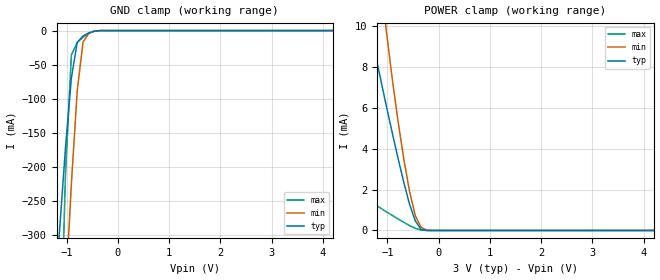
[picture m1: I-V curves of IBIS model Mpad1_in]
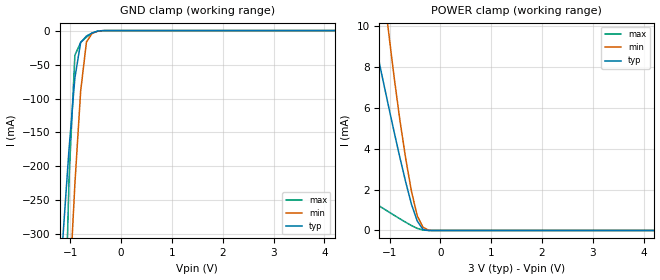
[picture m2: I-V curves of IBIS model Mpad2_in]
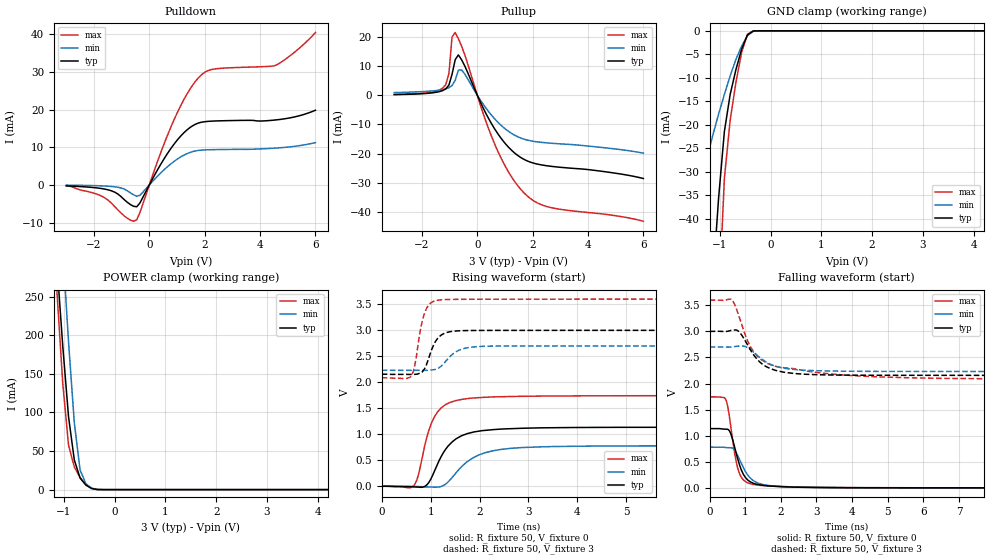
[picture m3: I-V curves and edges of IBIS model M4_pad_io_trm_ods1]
| Created by SiliconSmart  O-2018.09-SP2-3
[IBIS Ver]   4.0
[File Name]   as3316bc_rev1p3.ibs
[File Rev]   1.3
[Date]   Thursday Mar 21 2024
|[Source]   Avalanche Team
|[Notes]   Generated IBIS models from Silicon Smart
|[Rev 1.0]  Initial Release based on extracted netlist
|   Characterization
|[Rev 1.1]  Recharacterization with Hspice, run in high accuracy mode
|[Rev 1.2]  Recharacterization with Hspice, align with datasheet parameter
|[Rev 1.3]  Update the pin to the package pinout assignment
|[Disclaimer]   THE MODEL LIBRARIES ARE PROVIDED AS IS.
|[Copyright]   Copyright 2019, Avalanche Technology., All Rights Reserved
[Component]   as30xx316_BGA
[Manufacturer] Avalanche Technology
| CONTENT :
| This file contains IBIS MODEL for PSRAM device
| AS3001316, AS3004316, AS3008316, AS3016316
| USAGE :
| The models are derived for the 2.7V to 3.6V I/O Operation.
| Temperatures for model generation: typ: 25, max: -40, min: 105
| Voltages : typ: 3.0V, min: 2.7V, max: 3.6V
| PACKAGES SUPPORTED :
| 48-ball FBGA (10mm x 10mm)
| VERIFICATION
| Errors  : 0
| Warnings: 10
| All warnings due to non-monotonic data:
[Package]
R_pkg   0   0 0
L_pkg   0   0 0
C_pkg   0   0 0
[Pin]   signal_name   model_name R_pin   L_pin   C_pin
H6   ADDR_19   Mpad1_in   0.0752   1.401E-09   0.684E-12
H1   ADDR_18   Mpad1_in   0.1092   1.943E-09   0.751E-12
D3   ADDR_17   Mpad1_in   0.1463   2.505E-09   1.065E-12
E4   ADDR_16   Mpad1_in   0.1612   2.777E-09   1.167E-12
F4   ADDR_15   Mpad1_in   0.1337   2.362E-09   1.112E-12
F3   ADDR_14   Mpad1_in   0.1937   3.618E-09   1.182E-12
G4   ADDR_13   Mpad1_in   0.6132   9.666E-09   2.965E-12
G3   ADDR_12   Mpad1_in   0.5553   11.39E-09   2.992E-12
H5   ADDR_11   Mpad1_in   0.5095   10.54E-09   2.784E-12
H4   ADDR_10   Mpad1_in   0.5085   8.139E-09   2.608E-12
H3   ADDR_9   Mpad1_in   0.6314   8.467E-09   2.753E-12
H2   ADDR_8   Mpad1_in   0.6215   8.571E-09   2.739E-12
D4   ADDR_7   Mpad1_in   0.1869   2.994E-09   1.300E-12
C4   ADDR_6   Mpad1_in   0.1507   2.486E-09   1.156E-12
C3   ADDR_5   Mpad1_in   0.1641   2.806E-09   1.081E-12
B4   ADDR_4   Mpad1_in   0.2121   3.648E-09   1.267E-12
B3   ADDR_3   Mpad1_in   0.2174   3.718E-09   1.391E-12
A5   ADDR_2   Mpad1_in   0.2699   5.112E-09   1.665E-12
A4   ADDR_1   Mpad1_in   0.2419   4.762E-09   1.566E-12
A3   ADDR_0   Mpad1_in   0.2438   4.120E-09   1.508E-12
A2   G#   Mpad2_in   0.2799   4.414E-09   1.651E-12
B5   E#   Mpad2_in   0.1988   3.329E-09   1.209E-12
G5   W#   Mpad2_in   0.3304   4.956E-09   1.725E-12
B2   UB#   Mpad2_in   0.3210   5.026E-09   2.051E-12
A1   LB#   Mpad2_in   0.2761   4.637E-09   1.872E-12
G1   DQ_15   Mpad_io   0.0818   1.440E-09   0.758E-12
F1   DQ_14   Mpad_io   0.0722   1.269E-09   0.671E-12
F2   DQ_13   Mpad_io   0.1073   1.763E-09   0.829E-12
E2   DQ_12   Mpad_io   0.1038   1.649E-09   0.806E-12
D2   DQ_11   Mpad_io   0.1029   1.657E-09   0.819E-12
C2   DQ_10   Mpad_io   0.1069   1.768E-09   0.820E-12
C1   DQ_9   Mpad_io   0.0842   1.423E-09   0.731E-12
B1   DQ_8   Mpad_io   0.0865   1.515E-09   0.776E-12
G6   DQ_7   Mpad_io   0.2711   4.295E-09   1.572E-12
F6   DQ_6   Mpad_io   0.1981   3.065E-09   1.253E-12
F5   DQ_5   Mpad_io   0.2781   4.148E-09   1.750E-12
E5   DQ_4   Mpad_io   0.1116   1.847E-09   0.835E-12
D5   DQ_3   Mpad_io   0.1145   1.910E-09   0.901E-12
C6   DQ_2   Mpad_io   0.1632   2.557E-09   1.079E-12
C5   DQ_1   Mpad_io   0.1544   2.582E-09   1.063E-12
B6   DQ_0   Mpad_io   0.2212   3.537E-09   1.114E-12
D1   VSS   GND   NA   NA   NA
E6   VSS   GND   NA   NA   NA
D6   VCC   POWER   NA   NA   NA
E1   VCC   POWER   NA   NA   NA
| pad_io
[Model Selector] Mpad_io
| Model Description
M4_pad_io_trm_ods1   60 Ohms drv strength
| Models and submodels in the file (3): Mpad1_in (Input), Mpad2_in (Input), M4_pad_io_trm_ods1 (I/O)
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| pad1_in
[Model] Mpad1_in
Model_type Input
Enable   Active-High
Vinl  =  0.6
Vinh  =  2.4
| Capacitance  typ   min   max
C_comp   2.857182e-12   2.353202e-12   3.152994e-12
| Variables   typ   min   max
[GND Clamp Reference]   0   0   0
[POWER Clamp Reference]   3   2.7   3.6
[Pulldown Reference]   0   0   0
[Pullup Reference]   3   2.7   3.6
[Temperature Range]   25   105   -40
[Voltage Range]   3   2.7   3.6
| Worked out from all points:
|   GND clamp passes 1 mA (typ) near -0.47 V on its own axis
|   POWER clamp passes 1 mA (typ) near -0.53 V on its own axis
[GND Clamp]
| Voltage   I(typ)   I(min)   I(max)
-3V       -2.489A    -3.622A    -6.286A
-1.252V   -415.1mA   -737.7mA   -841.9mA
-1.138V   -289.6mA   -559.5mA   -509.9mA
-1.024V   -170.9mA   -387mA     -208.5mA
-910.3mV  -69.58mA   -225.3mA   -35.91mA
-796.6mV  -17.5mA    -88.85mA   -17.44mA
-682.8mV  -8.077mA   -16.84mA   -9.651mA
-569mV    -3.425mA   -3.886mA   -3.679mA
-455.2mV  -663.4uA   -928.9uA   -526.9uA
-227.6mV  -421.5nA   -3.52uA    -35.99nA
6V        0A         0A         0A
[POWER Clamp]
| Voltage   I(typ)   I(min)   I(max)
-3V       32.41mA    56.72mA    4.109mA
-1.366V   10.2mA     17.4mA     1.461mA
-1.252V   8.822mA    14.8mA     1.281mA
-1.024V   6.137mA    9.837mA    922.9uA
-910.3mV  4.838mA    7.526mA    746.6uA
-796.6mV  3.581mA    5.417mA    573.1uA
-682.8mV  2.387mA    3.545mA    403.9uA
-569mV    1.291mA    1.93mA     242.9uA
-455.2mV  467.9uA    721.2uA    103.5uA
-341.4mV  48.97uA    156.2uA    20.84uA
-113.8mV  7.993nA    354.4nA    880.4pA
6V        0A         0A         0A
| pad2_in
[Model] Mpad2_in
Model_type Input
Enable   Active-High
Vinl  =  0.6
Vinh  =  2.4
| Capacitance  typ   min   max
C_comp   2.865723e-12   2.362138e-12   3.161751e-12
| Variables   typ   min   max
[GND Clamp Reference]   0   0   0
[POWER Clamp Reference]   3   2.7   3.6
[Pulldown Reference]   0   0   0
[Pullup Reference]   3   2.7   3.6
[Temperature Range]   25   105   -40
[Voltage Range]   3   2.7   3.6
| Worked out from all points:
|   GND clamp passes 1 mA (typ) near -0.47 V on its own axis
|   POWER clamp passes 1 mA (typ) near -0.53 V on its own axis
[GND Clamp]
| Voltage   I(typ)   I(min)   I(max)
-3V       -2.583A    -3.873A    -6.564A
-1.138V   -296.1mA   -573.1mA   -531mA
-1.024V   -173.3mA   -391.8mA   -216.6mA
-910.3mV  -69.77mA   -226.3mA   -36.44mA
-796.6mV  -17.49mA   -89.03mA   -17.43mA
-682.8mV  -8.073mA   -16.84mA   -9.646mA
-569mV    -3.423mA   -3.884mA   -3.677mA
-455.2mV  -662.9uA   -928.4uA   -526.4uA
-227.6mV  -421nA     -3.517uA   -35.92nA
6V        0A         0A         0A
[POWER Clamp]
| Voltage   I(typ)   I(min)   I(max)
-3V       32.41mA    56.72mA    4.109mA
-1.366V   10.2mA     17.4mA     1.461mA
-1.252V   8.822mA    14.8mA     1.281mA
-1.024V   6.137mA    9.837mA    922.9uA
-910.3mV  4.838mA    7.526mA    746.6uA
-796.6mV  3.581mA    5.417mA    573.1uA
-682.8mV  2.387mA    3.545mA    403.9uA
-569mV    1.291mA    1.93mA     242.9uA
-455.2mV  467.9uA    721.2uA    103.5uA
-341.4mV  48.97uA    156.2uA    20.84uA
-113.8mV  7.993nA    354.4nA    880.4pA
6V        0A         0A         0A
[Model] M4_pad_io_trm_ods1
Model_type I/O
Enable   Active-High
Vinl  =  0.6
Vinh  =  2.4
Vmeas =  1.5
Cref  =  30e-12
| Capacitance  typ   min   max
C_comp   4.118801e-12   3.947848e-12   4.414159e-12
| Variables   typ   min   max
[GND Clamp Reference]   0   0   0
[POWER Clamp Reference]   3   2.7   3.6
[Pulldown Reference]   0   0   0
[Pullup Reference]   3   2.7   3.6
[Temperature Range]   25   105   -40
[Voltage Range]   3   2.7   3.6
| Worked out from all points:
|   slope of the pulldown table from 0 to 0.45 V, typ, clamps not added: 75.6 ohm
|   slope of the pullup table from 0 to 0.45 V, typ, clamps not added: 51.8 ohm
|   GND clamp passes 1 mA (typ) near -0.46 V on its own axis
|   POWER clamp passes 1 mA (typ) near -0.42 V on its own axis
|   falling waveform, R_fixture 50, V_fixture 0: 20-80 % time 325ps typ, 411ps min, 252ps max; typ from 1.14 V to 0 V
|   falling waveform, R_fixture 50, V_fixture 3: 20-80 % time 602ps typ, 661ps min, 794ps max; typ from 3 V to 2.15 V
|   rising waveform, R_fixture 50, V_fixture 0: 20-80 % time 466ps typ, 621ps min, 335ps max; typ from 0 V to 1.14 V
|   rising waveform, R_fixture 50, V_fixture 3: 20-80 % time 225ps typ, 326ps min, 176ps max; typ from 2.15 V to 3 V
[GND Clamp]
| Voltage   I(typ)   I(min)   I(max)
-3V       -379.8mA   -106mA     -725.8mA
-1.593V   -131.7mA   -42.01mA   -247mA
-1.479V   -111.8mA   -36.94mA   -208.5mA
-1.138V   -53.52mA   -22.25mA   -94.22mA
-1.024V   -35.67mA   -17.76mA   -59.08mA
-910.3mV  -21.49mA   -13.58mA   -31.51mA
-796.6mV  -13.6mA    -9.604mA   -19.09mA
-682.8mV  -8.279mA   -6.099mA   -11mA
-569mV    -3.88mA    -3.236mA   -4.53mA
-455.2mV  -866.7uA   -1.043mA   -727.1uA
-341.4mV  -35.72uA   -109.2uA   -11.2uA
6V        0A         0A         0A
[POWER Clamp]
| Voltage   I(typ)   I(min)   I(max)
-3V       2.191A     2.679A     2.475A
-1.138V   291mA      439mA      255.8mA
-1.024V   186.1mA    312.2mA    137.6mA
-910.3mV  94.47mA    191.5mA    57.5mA
-796.6mV  38.47mA    86.67mA    29.42mA
-682.8mV  15.04mA    25.47mA    15.61mA
-569mV    5.939mA    7.524mA    6.125mA
-455.2mV  1.483mA    1.86mA     1.35mA
-227.6mV  1.148uA    12.93uA    332nA
6V        0A         0A         0A
[Pulldown]
| Voltage   I(typ)   I(min)   I(max)
-3V       -248.9uA   -57.27uA   -211.8uA
-1.934V   -763.9uA   -203.6uA   -2.351mA
-1.479V   -1.326mA   -352.6uA   -4.122mA
-796.6mV  -4.614mA   -1.551mA   -8.859mA
-455.2mV  -5.81mA    -3.008mA   -9.281mA
413.8mV   5.511mA    3.198mA    8.617mA
827.6mV   10.2mA     5.892mA    16.24mA
1.345V    14.53mA    8.266mA    23.98mA
1.759V    16.42mA    9.161mA    28.37mA
2.276V    16.97mA    9.375mA    30.72mA
4.614V    17.32mA    9.818mA    31.97mA
6V        19.86mA    11.25mA    40.51mA
[Pullup]
| Voltage   I(typ)   I(min)   I(max)
-3V       187.4uA    871.4uA    220.3uA
-1.252V   1.555mA    1.876mA    2.377mA
-1.024V   3.43mA     2.541mA    7.364mA
-910.3mV  7.139mA    3.267mA    19.92mA
-796.6mV  12.13mA    5.096mA    21.41mA
-682.8mV  13.76mA    8.544mA    19.32mA
-569mV    12.16mA    8.636mA    16.81mA
620.7mV   -11.43mA   -8.01mA    -16.55mA
1.138V    -17.91mA   -12.44mA   -26.44mA
1.655V    -21.81mA   -14.96mA   -33.11mA
2.586V    -24.25mA   -16.39mA   -38.3mA
6V        -28.52mA   -19.85mA   -43.17mA
[Ramp]
dV/dt_r   0.681951/0.465717n  0.468514/0.620601n  1.04707/0.335033n
dV/dt_f   0.507478/0.602469n  0.281038/0.661038n  0.908676/0.793971n
R_load = 50
[Falling Waveform]
R_fixture = 50
V_fixture = 0
V_fixture_min = 0
V_fixture_max = 0
| Time   V(typ)   V(min)   V(max)
0s        1.137V     780.9mV    1.745V
449.9ps   1.126V     772.6mV    1.697V
508.1ps   1.122V     771mV      1.558V
603.1ps   1.02V      768.8mV    1.127V
721ps     726.5mV    702.8mV    590.2mV
828.5ps   459.1mV    557.6mV    291.5mV
1.004ns   198.3mV    313.9mV    120.4mV
1.349ns   64.63mV    94.58mV    52.82mV
3.774ns   2.102mV    4.005mV    6.578mV
21.88ns   -42.85nV   140nV      61.39nV
[Falling Waveform]
R_fixture = 50
V_fixture = 3
V_fixture_min = 2.7
V_fixture_max = 3.6
| Time   V(typ)   V(min)   V(max)
0s        3V         2.7V       3.6V
634.8ps   3.023V     2.703V     3.597V
847.3ps   2.977V     2.719V     3.241V
1.169ns   2.619V     2.638V     2.678V
1.378ns   2.432V     2.516V     2.503V
1.62ns    2.314V     2.399V     2.386V
2.203ns   2.207V     2.282V     2.298V
3.494ns   2.163V     2.239V     2.178V
7.486ns   2.158V     2.232V     2.093V
21.88ns   2.154V     2.232V     2.086V
[Rising Waveform]
R_fixture = 50
V_fixture = 0
V_fixture_min = 0
V_fixture_max = 0
| Time   V(typ)   V(min)   V(max)
0s        24.24nV    299.5nV    41.88nV
653.2ps   -9.927mV   -1.656mV   10.12mV
759.1ps   -16.54mV   -3.819mV   256.1mV
919.1ps   24.84mV    -9.607mV   933.3mV
1.136ns   419.1mV    -14.93mV   1.424V
1.43ns    847.3mV    159.7mV    1.625V
1.82ns    1.031V     521.5mV    1.695V
2.443ns   1.101V     711mV      1.724V
3.955ns   1.132V     771.8mV    1.74V
21.88ns   1.137V     780.9mV    1.745V
[Rising Waveform]
R_fixture = 50
V_fixture = 3
V_fixture_min = 2.7
V_fixture_max = 3.6
| Time   V(typ)   V(min)   V(max)
0s        2.154V     2.232V     2.086V
596.6ps   2.152V     2.231V     2.111V
670.7ps   2.154V     2.231V     2.302V
806.3ps   2.186V     2.231V     3.083V
893ps     2.296V     2.231V     3.375V
1.061ns   2.72V      2.243V     3.558V
1.23ns    2.917V     2.326V     3.588V
1.576ns   2.991V     2.616V     3.596V
2.22ns    2.998V     2.696V     3.598V
21.88ns   3V         2.7V       3.6V
